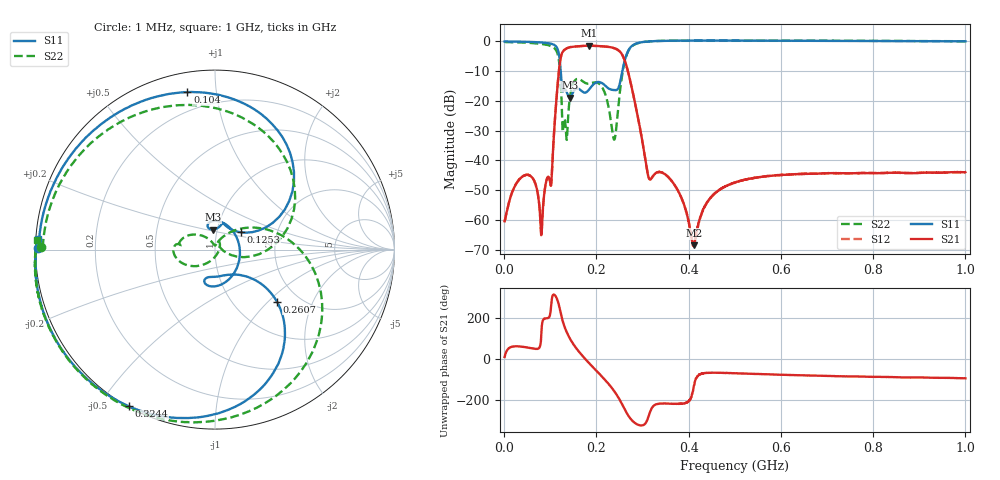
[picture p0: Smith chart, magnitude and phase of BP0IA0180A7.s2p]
!Agilent Technologies,E8358A,US41080443,A.07.50.56
!Agilent E8358A: A.07.50.56
!Date: Tuesday, October 31, 2017 22:09:42
!Correction: S11(Full 2 Port(1,2))
!S21(Full 2 Port(1,2))
!S12(Full 2 Port(1,2))
!S22(Full 2 Port(1,2))
!S2P File: Measurements: S11, S21, S12, S22:
# Hz S  dB  R 50
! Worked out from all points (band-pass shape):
!   1601 points, 1 MHz to 1 GHz, reference 50 ohm
!   highest |S21| = -1.56 dB at 183.3 MHz (marker M1); lowest = -68.5 dB at 411.8 MHz (marker M2)
!   |S21| within 3 dB of the highest: 124.3 MHz to 255.9 MHz (131.6 MHz wide, 69.2 % of centre)
!   lowest |S11| = -19.0 dB at 142.1 MHz (marker M3), VSWR 1.25, Z = 47.7 + j10.8 ohm
!   |S11| at or under -10 dB: 122.7 MHz to 256.4 MHz (133.7 MHz wide, 70.6 % of centre)
!   |S22| runs from -33.1 to 0.2 dB; largest |S21 - S12| = 0.0047
!   S11 on the Smith chart (normalised r, x): 1 MHz: 0.01, +0.00; 104 MHz: 0.10, +0.84; 125.3 MHz: 1.31, +0.26; 260.7 MHz: 1.55, -1.13; 324.4 MHz: 0.00, -0.59; 1 GHz: 0.01, +0.03
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1000000  -0.14 179.5  -60.38 10.8  -60.38 11.7  -0.29 179.2
4.907688e7  -0.27 156.2  -44.83 57.3  -44.79 58.2  -0.55 156.2
8.092e7  -0.49 132.9  -64.76 134.0  -64.49 134.0  -0.95 132.3
1.040219e8  -1.01 99.9  -42.52 -57.1  -42.49 -57.1  -1.87 95.8
1.171338e8  -3.34 52.0  -12.55 -82.1  -12.53 -81.9  -5.07 37.2
1.252506e8  -15.17 33.4  -4.14 -159.1  -4.13 -158.9  -23.15 -16.6
1.321188e8  -16.24 74.1  -2.79 151.5  -2.77 151.6  -26.85 54.7
1.421088e8  -18.98 95.8  -2.10 103.0  -2.08 103.1  -19.46 -128.0
1.677081e8  -16.69 53.4  -1.68 21.7  -1.67 21.6  -13.20 172.5
1.833175e8  -16.39 -29.9  -1.56 -17.5  -1.57 -17.6  -14.29 174.6
2.126631e8  -14.14 -106.4  -1.76 -86.4  -1.80 -86.4  -15.53 151.8
2.382625e8  -16.41 -87.0  -2.37 -155.3  -2.40 -155.3  -33.02 91.1
2.6074e8  -6.92 -40.0  -6.20 117.4  -6.27 117.6  -7.34 5.5
2.863394e8  -0.84 -87.8  -22.69 43.4  -22.70 43.9  -0.92 -71.9
3.244262e8  -0.04 -118.7  -44.91 132.4  -44.93 132.3  -0.04 -112.1
3.344162e8  0.02 -123.4  -43.92 141.6  -43.87 141.9  0.03 -117.8
4.118388e8  0.16 -145.1  -68.48 -127.1  -68.55 -127.1  0.18 -143.0
4.4056e8  0.16 -149.8  -53.86 -67.0  -53.92 -66.8  0.18 -148.3
5.005e8  0.15 -157.2  -47.44 -68.9  -47.41 -68.6  0.17 -156.2
6.672081e8  0.09 -169.9  -44.48 -80.2  -44.47 -79.8  0.12 -169.4
8.339162e8  0.00 -177.6  -44.13 -87.5  -44.15 -87.5  0.03 -177.3
1e9  -0.10 176.6  -43.94 -93.6  -44.01 -93.3  -0.07 177.0
